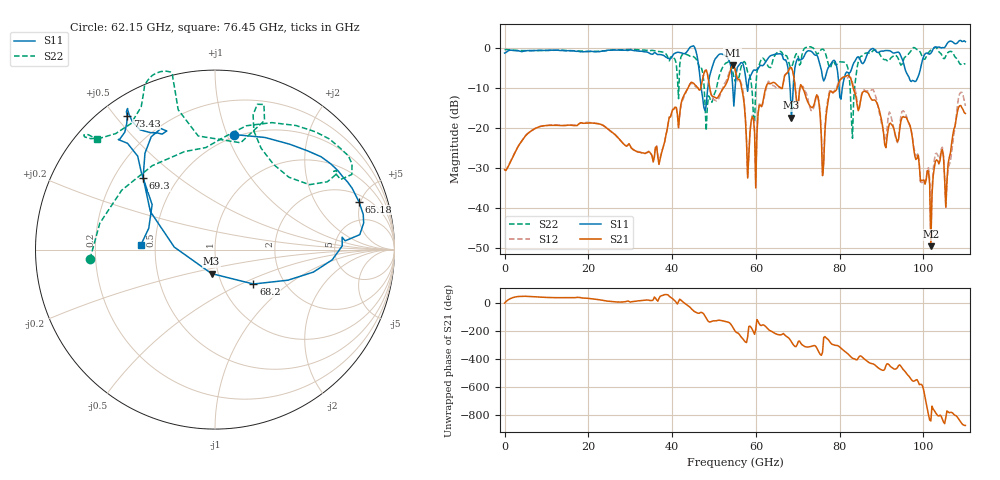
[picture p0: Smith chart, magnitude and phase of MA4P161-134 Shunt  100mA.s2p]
!Keysight Technologies,N5247B,US61255204,A.15.70.20
!Date: Friday, October 21, 2022 14:16:22
!Correction: S11(C  4-Port  )
!S31(C  4-Port  )
!S13(C  4-Port  )
!S33(C  4-Port  )
!S2P File: Measurements: S11, S31, S13, S33:
# Hz S  dB  R 50
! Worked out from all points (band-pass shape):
!   401 points, 10 MHz to 110 GHz, reference 50 ohm
!   highest |S21| = -4.29 dB at 54.46 GHz (marker M1); lowest = -49.5 dB at 101.8 GHz (marker M2)
!   |S21| within 3 dB of the highest: 53.48 GHz to 55.47 GHz (1.994 GHz wide, 3.66 % of centre); 66.77 GHz to 69.05 GHz (2.279 GHz wide, 3.36 % of centre)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
!   lowest |S11| = -17.4 dB at 68.48 GHz (marker M3), VSWR 1.31, Z = 46.5 - j12.6 ohm
!   |S11| at or under -10 dB: 46.95 GHz to 48.51 GHz (1.564 GHz wide, 3.28 % of centre); 68.14 GHz to 68.9 GHz (760.6 MHz wide, 1.11 % of centre); 79.86 GHz to 80.62 GHz (765.2 MHz wide, 0.954 % of centre)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
!   |S22| runs from -22.6 to 0.3 dB; largest |S21 - S12| = 0.16
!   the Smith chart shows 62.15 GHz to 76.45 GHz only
!   S11 on the Smith chart (normalised r, x): 62.15 GHz: 0.48, +1.06; 65.18 GHz: 2.58, +4.83; 68.2 GHz: 1.40, -0.59; 69.3 GHz: 0.32, +0.38; 73.43 GHz: 0.07, +0.54; 76.45 GHz: 0.41, +0.02
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1e7  -1.26 -180.0  -30.41 -0.9  -30.40 -1.1  -0.38 179.9
1.843332e10  -0.91 130.9  -18.70 35.8  -18.71 35.7  -0.75 140.7
3.685665e10  -1.62 126.7  -29.08 32.2  -28.93 32.3  -0.85 134.1
4.565585e10  -0.66 52.9  -9.39 -66.8  -9.76 -65.3  -2.68 28.0
4.84056e10  -10.96 139.0  -6.37 -121.7  -6.26 -121.4  -14.59 130.6
5.445505e10  -9.58 97.7  -4.29 -172.2  -4.35 -172.0  -5.78 127.8
5.5005e10  -10.48 -177.8  -5.19 160.4  -5.39 160.0  -8.27 147.1
5.802972e10  -10.82 160.8  -32.50 117.4  -32.28 116.9  -6.04 167.7
6.215435e10  -3.75 80.7  -10.75 -163.6  -11.47 -158.2  -3.11 -175.6
6.517908e10  -1.46 18.4  -9.37 134.6  -10.09 160.9  -1.04 44.0
6.82038e10  -10.84 -41.9  -4.82 95.4  -4.99 92.4  -4.79 44.4
6.847878e10  -17.40 -98.2  -4.93 82.2  -5.13 79.7  -4.79 55.5
6.93037e10  -4.94 135.0  -9.29 49.4  -9.04 48.8  -2.15 74.2
7.342832e10  -1.01 123.3  -14.88 52.2  -15.71 50.4  0.14 111.6
7.645305e10  -7.65 176.6  -21.19 119.5  -20.20 131.4  -0.92 136.9
8.085265e10  -8.55 -75.9  -7.26 23.0  -7.67 23.3  -3.50 -143.8
8.305245e10  -4.49 -45.4  -9.18 -34.9  -8.65 -18.9  -22.56 23.4
8.607718e10  -2.94 6.5  -10.84 -45.3  -10.69 -44.3  -1.30 -14.2
9.185165e10  -0.66 72.0  -18.93 -84.0  -15.98 -80.9  -3.04 67.0
9.762612e10  -8.19 176.6  -24.86 160.7  -24.38 159.0  0.13 166.4
1.017508e11  -1.31 -88.2  -49.51 -123.2  -48.27 -116.1  -0.55 -124.2
1.1e11  1.57 9.0  -16.35 -155.2  -14.43 -160.0  -4.04 15.7
